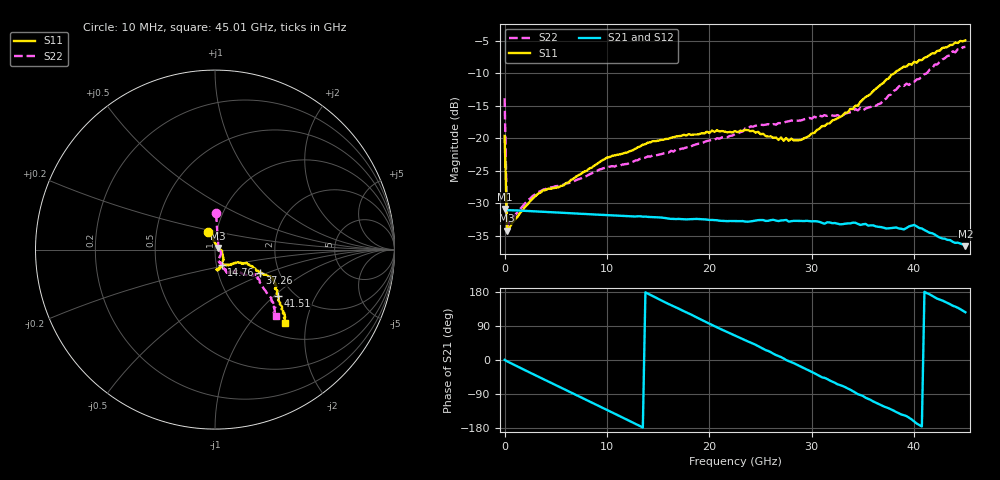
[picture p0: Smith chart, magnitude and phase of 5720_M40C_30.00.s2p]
! Device:  ADRF5720
! Description: 0.5dB LSB GaAs MMIC 6-bit Digital Attenuator
! Frequency:  0.000009 -  40 GHz
! Ports:
!	RF1	= Port 1
!	RF2	= Port 2
! Vdd:  3.3 Volt
! Vss:  -3.3 Volt
! Control:  0/3.3 Volt
! State:  30.00 dB attenuation
! Data:  The device was measured using G-S-G Probes on a matrix board.
!  Data was collected using an calibrated 4 port network analyzer.
!  The reference plane for this measurement is at the launchers.
! Note:  Analog Devices supplies this data as a sample of measured data
!  for this product.  Your particular data for this product may vary.
!  Data was taken at -40 degrees C.
!  Analog Devices reserves the right to change this data at anytime.
# GHZ S DB R 45.0
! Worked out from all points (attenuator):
!   181 points, 10 MHz to 45.01 GHz, reference 45 ohm
!   highest |S21| = -30.87 dB at 10 MHz (marker M1); lowest = -36.6 dB at 45.01 GHz (marker M2)
!   lowest |S11| = -34.2 dB at 260 MHz (marker M3), VSWR 1.04, Z = 46.5 + j0.9 ohm
!   |S11| at or under -10 dB: start of sweep to 38.07 GHz
!   |S22| runs from -33.6 to -6.0 dB; largest |S21 - S12| = 0.00016
!   S11 on the Smith chart (normalised r, x): 10 MHz: 0.91, +0.18; 14.76 GHz: 1.06, -0.19; 37.26 GHz: 1.59, -0.45; 41.51 GHz: 1.66, -1.06; 45.01 GHz: 1.27, -1.51
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0.01  -19.64 110.8  -30.87 0.4  -30.89 0.4  -13.86 88.4
0.26  -34.21 29.8  -31.05 -3.6  -31.07 -3.7  -33.56 23.0
3.26  -28.54 -7.6  -31.26 -43.5  -31.28 -43.5  -28.28 -28.5
5.76  -27.27 -23.4  -31.46 -76.2  -31.48 -76.2  -27.15 -47.9
7.76  -25.14 -37.8  -31.63 -102.3  -31.65 -102.3  -25.94 -62.1
10.01  -22.98 -47.9  -31.83 -131.8  -31.85 -131.9  -24.47 -68.2
14.76  -20.45 -66.6  -32.16 164.9  -32.17 164.8  -22.64 -70.4
15.26  -20.26 -68.3  -32.18 158.0  -32.20 157.9  -22.47 -70.5
20.26  -18.82 -81.6  -32.56 92.5  -32.58 92.4  -20.26 -64.6
22.76  -19.06 -85.3  -32.74 61.2  -32.76 61.2  -19.30 -65.4
24.01  -18.92 -80.8  -32.78 46.4  -32.80 46.3  -18.20 -64.0
27.76  -20.40 -68.3  -32.82 -2.8  -32.85 -2.9  -17.39 -61.5
30.26  -19.18 -48.8  -32.75 -34.8  -32.77 -35.0  -16.69 -61.9
32.76  -16.75 -29.2  -33.23 -66.2  -33.26 -66.4  -16.66 -55.5
36.26  -12.41 -25.6  -33.55 -112.5  -33.57 -112.5  -15.03 -43.2
37.26  -10.99 -27.6  -33.87 -124.8  -33.88 -125.0  -13.93 -41.8
37.76  -10.28 -27.2  -33.81 -130.4  -33.84 -130.5  -13.27 -40.0
38.76  -9.25 -25.9  -33.92 -143.9  -33.92 -144.2  -11.80 -35.0
40.01  -8.25 -29.3  -33.33 -162.3  -33.34 -162.5  -11.32 -32.5
41.51  -7.20 -36.2  -34.53 173.5  -34.58 173.1  -9.46 -37.9
43.76  -5.65 -42.4  -35.91 143.3  -35.90 143.1  -6.64 -43.7
45.01  -4.97 -46.3  -36.59 126.0  -36.63 126.0  -5.96 -47.6
